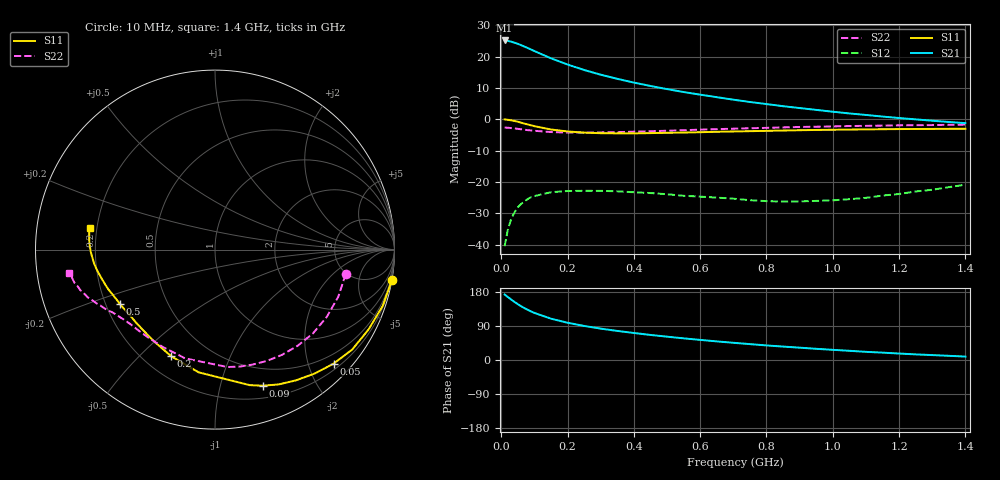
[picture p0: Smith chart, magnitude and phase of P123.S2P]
! Date: Tue Aug 08 08:14:29 1995
# MHZ  S  MA  R  50.0000
!  POLYFET RF DEVICES
!  P123
!  S PARAMETERS
!  VDS=12.5V, IDQ=200mA
!FREQ  S11MAG S11ANG S21MAG S21ANG S12MAG S12ANG S22MAG S22ANG
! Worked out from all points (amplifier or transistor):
!   36 points, 10 MHz to 1.4 GHz, reference 50 ohm
!   highest |S21| = 25.2 dB at 10 MHz (marker M1)
!   |S21| within 3 dB of that: start of sweep to 92.01 MHz
!   unconditionally stable (mu >= 1): 749 MHz to 1.185 GHz
!   at 70 MHz: K = 0.08, MSG = 24.7 dB, |S12| = -26.2 dB
!   at 550 MHz: K = 0.70, MSG = 16.6 dB, |S12| = -24.4 dB
!   at 1.4 GHz: K = 0.73, MSG = 9.8 dB, |S12| = -20.8 dB
!   S11 on the Smith chart (normalised r, x): 10 MHz: -0, -12; 50 MHz: 0.31, -2.45; 90 MHz: 0.32, -1.37; 200 MHz: 0.31, -0.63; 500 MHz: 0.26, -0.25; 1.4 GHz: 0.17, +0.08
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10  1.001 -9.6  18.22 172.8  0.00946 90.2  0.7406 -10.7
20  0.9856 -18.6  17.9 166.0  0.01762 77.6  0.7354 -20.9
30  0.9644 -27.4  17.4 159.4  0.02591 71.6  0.7269 -31.0
40  0.946 -36.0  16.78 153.1  0.03291 66.2  0.7183 -40.5
50  0.9168 -43.9  16.08 147.2  0.03953 59.6  0.7065 -49.3
60  0.8858 -51.3  15.32 141.8  0.04475 54.9  0.6952 -57.5
70  0.8565 -58.3  14.52 136.8  0.04924 50.3  0.6842 -65.0
80  0.831 -64.6  13.78 132.3  0.05366 46.7  0.6739 -72.0
90  0.8046 -70.5  13.05 128.1  0.05742 42.4  0.6662 -78.1
100  0.7794 -75.7  12.32 124.2  0.05975 39.1  0.6578 -83.9
150  0.6899 -97.6  9.449 109.0  0.0688 26.5  0.6286 -105.3
200  0.6424 -112.3  7.515 98.3  0.07184 18.4  0.6155 -118.5
250  0.6148 -123.1  6.153 89.9  0.07259 12.7  0.6151 -127.5
300  0.6022 -131.0  5.172 82.8  0.07235 8.1  0.6204 -133.5
350  0.5992 -137.2  4.445 76.7  0.07112 5.2  0.6266 -138.0
400  0.5986 -142.3  3.868 71.3  0.06862 2.9  0.6368 -141.6
500  0.6106 -150.4  3.046 61.6  0.06386 -0.2  0.659 -146.7
600  0.6246 -156.8  2.484 53.0  0.05849 0.0  0.687 -150.5
750  0.6488 -164.8  1.898 41.9  0.05129 5.2  0.723 -155.4
950  0.6785 -173.6  1.42 29.5  0.04999 21.7  0.7644 -160.7
1200  0.7009 177.1  1.052 17.0  0.06442 41.2  0.8045 -166.8
1400  0.7079 170.4  0.8726 9.0  0.09074 48.1  0.8257 -170.8
